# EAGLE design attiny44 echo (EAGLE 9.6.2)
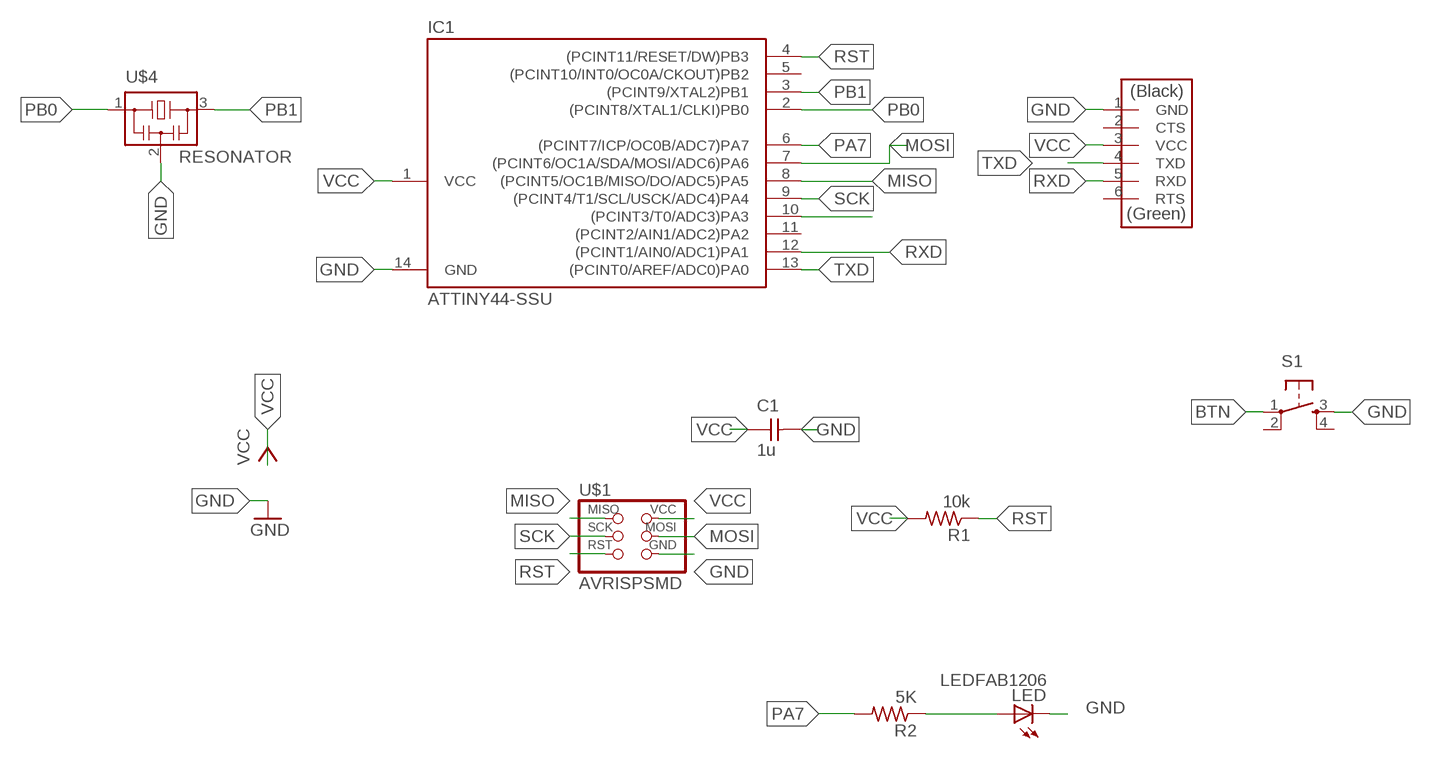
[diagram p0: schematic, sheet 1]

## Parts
C1  1u  CAP-UNPOLARIZEDFAB  [C1206FAB]
IC1  ATTINY44-SSU  [SOIC14]
LED  LEDFAB1206  [LED1206FAB]
R1  10k  RES-US1206FAB  [R1206FAB]
R2  5K  RES-US1206FAB  [R1206FAB]
S1  6MM_SWITCH6MM_SWITCH  [6MM_SWITCH]
U$1  AVRISPSMD  [2X03SMD]
U$4  RESONATOR  [EFOBM]
U$5  FTDI-SMD-HEADER  [1X06SMD]

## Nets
BTN: IC1.10((PCINT3/T0/ADC3)PA3) S1.1(P)
GND: C1.2 IC1.14(GND) LED.2(C) S1.3(S) U$1.6(GND) U$4.2 U$5.1(GND)
MISO: IC1.8((PCINT5/OC1B/MISO/DO/ADC5)PA5) U$1.1(MISO)
MOSI: IC1.7((PCINT6/OC1A/SDA/MOSI/ADC6)PA6) U$1.4(MOSI)
N$1: LED.1(A) R2.1
PA7: IC1.6((PCINT7/ICP/OC0B/ADC7)PA7) R2.2
PB0: IC1.2((PCINT8/XTAL1/CLKI)PB0) U$4.1
PB1: IC1.3((PCINT9/XTAL2)PB1) U$4.3
RST: IC1.4((PCINT11/RESET/DW)PB3) R1.1 U$1.5(RST)
RXD: IC1.12((PCINT1/AIN0/ADC1)PA1) U$5.5(RXD)
SCK: IC1.9((PCINT4/T1/SCL/USCK/ADC4)PA4) U$1.3(SCK)
TXD: IC1.13((PCINT0/AREF/ADC0)PA0) U$5.4(TXD)
VCC: C1.1 IC1.1(VCC) R1.2 U$1.2(VCC) U$5.3(VCC)
Unconnected: IC1.5((PCINT10/INT0/OC0A/CKOUT)PB2) IC1.11((PCINT2/AIN1/ADC2)PA2) S1.2(P1) S1.4(S1) U$5.2(CTS) U$5.6(RTS)

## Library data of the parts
C1 = fab:CAP-UNPOLARIZED
IC1 = fab:ATTINY44
LED = fab:LED: LED
R1 R2 = fab:RES-US: Resistor (US Symbol)
S1 = fab:6MM_SWITCH: OMRON SWITCH
U$1 = fab:AVRISP
U$4 = fab:RESONATOR
U$5 = fab:FTDI-SMD-HEADER

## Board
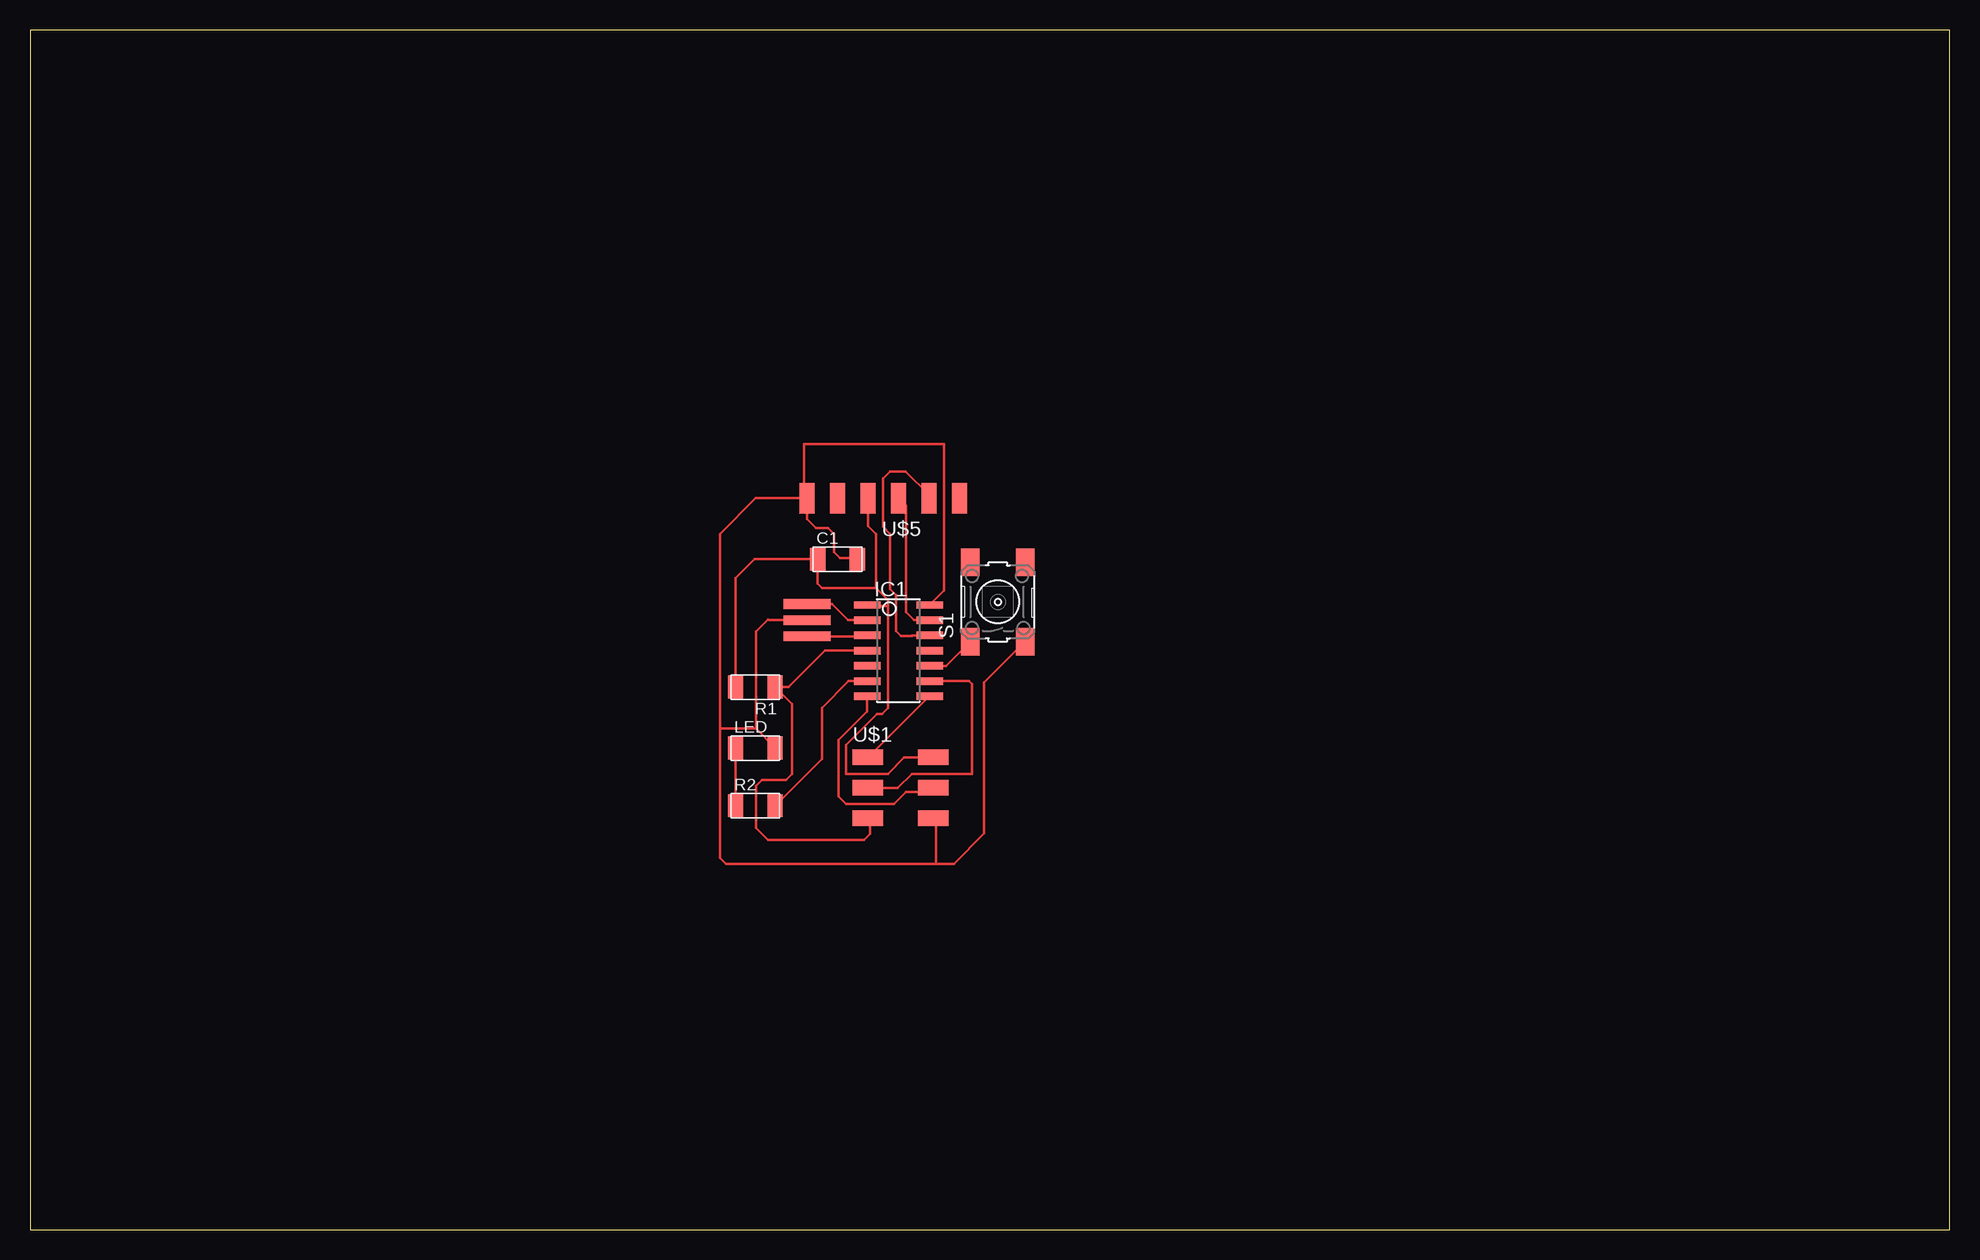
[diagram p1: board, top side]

Size 160 x 100 mm. Coordinates in mm from the lower left corner, seen from the top.
Outline: 0,0 160,0 160,100 0,100 0,0
Copper layers (1*16): Top 0.035mm / dielectric 1.5mm / Bottom 0.035mm
Design rules "default *": minimum track width 8mil, minimum drill 0.35mm, track to track 16mil, track to pad 16mil, pad to pad 6mil, via to via 6mil, smd to smd 16mil, copper to edge 40mil, drill to drill 6mil, minimum pad ring 10mil, minimum via ring 8mil, stop-mask expansion 4mil, vias tented up to drill 0mil, thermal gap 10mil

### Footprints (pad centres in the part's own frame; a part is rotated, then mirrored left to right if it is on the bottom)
C1206FAB = smd 1.27 x 1.905: 1 -1.651,0; 2 1.651,0
SOIC14 = smd 0.61 x 2.21: 1 -3.81,-2.603; 2 -2.54,-2.603; 3 -1.27,-2.603; 4 0,-2.603; 5 1.27,-2.603; 6 2.54,-2.603; 7 3.81,-2.603; 8 3.81,2.603; 9 2.54,2.603; 10 1.27,2.603; 11 0,2.603; 12 -1.27,2.603; 13 -2.54,2.603; 14 -3.81,2.603
LED1206FAB = smd 1.27 x 1.905: 1 -1.651,0; 2 1.651,0
R1206FAB = smd 1.27 x 1.905: 1 -1.651,0; 2 1.651,0
6MM_SWITCH = smd 2.286 x 1.524: 1 -3.302,2.286; 2 3.302,2.286; 3 -3.302,-2.286; 4 3.302,-2.286
2X03SMD = smd 2.54 x 1.27: 1 -2.54,2.54; 2 2.92,2.54; 3 -2.54,0; 4 2.92,0; 5 -2.54,-2.54; 6 2.92,-2.54
EFOBM = smd 0.8 x 3.9: 1 -1.35,0; 2 0,0; 3 1.35,0
1X06SMD = smd 2.54 x 1.27: 1 0,6.35; 2 0,3.81; 3 0,1.27; 4 0,-1.27; 5 0,-3.81; 6 0,-6.35

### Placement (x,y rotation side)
C1  67.31,55.88 0 top
IC1  72.39,48.26 270 top
LED  60.46,40.14 0 top
R1  60.46,45.22 180 top
R2  60.46,35.33 0 top
S1  80.67,52.32 90 top
U$1  72.39,36.83 0 top
U$4  64.77,50.8 270 top
U$5  71.12,60.96 90 top

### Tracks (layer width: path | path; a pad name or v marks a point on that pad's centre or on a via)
BTN
  Top 0.203: S1.1 76.36,46.99 IC1.10
GND
  Top 0.203: U$4.2 61.59,50.8 61.52,50.86 60.5,49.84 60.5,41.75 | LED.2 60.5,41.75 | 60.5,41.75 57.5,41.75 | 57.5,41.75 57.5,31 58,30.5 75.5,30.5 | 75.5,30.5 75.5,34.1 U$1.6 | 75.5,30.5 77,30.5 79.53,33.03 79.53,45.59 S1.3 | 57.5,41.75 57.5,58 60.46,60.96 U$5.1 | C1.2 68.84,56 67.5,56 67,56.5 67,58 66.5,58.5 65.5,58.5 64.77,59.23 U$5.1 | IC1.14 76.2,53.28 76.2,65.5 64.5,65.5 64.5,61.23 U$5.1
MISO
  Top 0.203: U$1.1 74.93,44.45 IC1.8
MOSI
  Top 0.203: U$1.4 74.98,36.5 73,36.5 72,35.5 68,35.5 67.39,36.11 67.39,40.8 69.79,43.2 IC1.7
N$1
  Top 0.203: R2.1 LED.1
PA7
  Top 0.203: R2.2 66,39.22 66,43.5 68.22,45.72 IC1.6
PB0
  Top 0.203: U$4.1 66.85,52.15 68.2,50.8 IC1.2
PB1
  Top 0.203: U$4.3 69.71,49.45 IC1.3
RST
  Top 0.203: U$1.5 70,34.14 70,33 69.5,32.5 61.5,32.5 60.5,33.5 60.5,37 61,37.5 63,37.5 63.5,38 63.5,43.83 R1.1 63.22,45.22 66.26,48.26 IC1.4
RXD
  Top 0.203: U$5.5 74.93,61.26 72.99,63.2 71.7,63.2 71.1,62.6 71.1,58.6 71.7,58 71.7,53.4 72.2,52.9 72.2,49.9 72.6,49.5 73.5,49.5 73.53,49.53 IC1.12
SCK
  Top 0.203: IC1.9 78.28,45.72 78.5,45.5 78.5,38 73.5,38 72.33,36.83 U$1.3
TXD
  Top 0.203: U$5.4 73,60.35 73,51.5 73.7,50.8 IC1.13
VCC
  Top 0.203: U$1.2 72.87,39.37 71.5,38 68,38 68,40.4 70.6,43 71,43 71.5,43.5 71.5,52 | IC1.1 69.86,52 71.5,52 | 71.5,52 71.5,52.5 70.5,53.5 | 70.5,53.5 66,53.5 65.66,53.84 C1.1 60.38,55.88 58.81,54.31 R1.2 | 70.5,53.5 70.5,58 69.85,58.65 U$5.3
